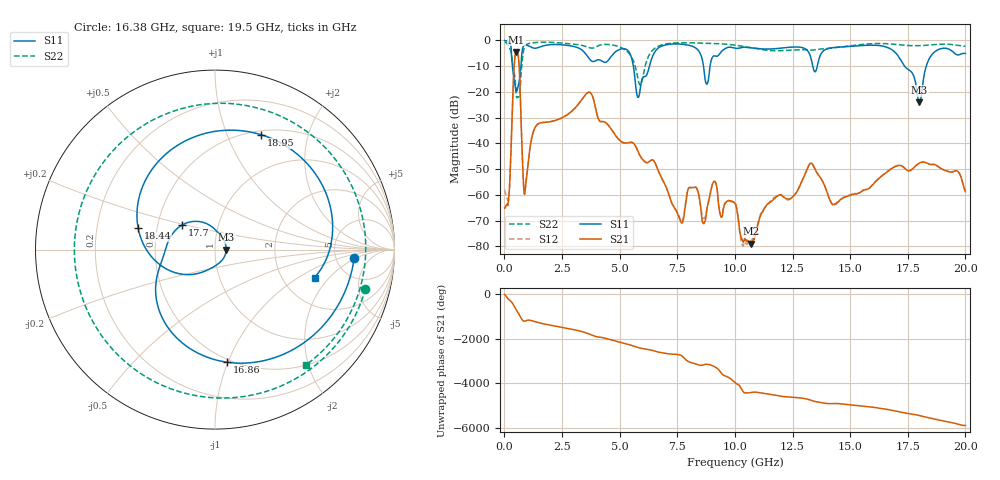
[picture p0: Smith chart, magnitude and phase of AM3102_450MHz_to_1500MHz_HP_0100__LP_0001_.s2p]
!Agilent Technologies,E8364B,MY43040894,A.07.50.67
!Agilent E8364B: A.07.50.67
!Date: Thursday, January 11, 2018 05:34:59
!Correction: S11(Full 2 Port(1,2))
!S21(Full 2 Port(1,2))
!S12(Full 2 Port(1,2))
!S22(Full 2 Port(1,2))
!S2P File: Measurements: S11, S21, S12, S22:
# Hz S  dB  R 50
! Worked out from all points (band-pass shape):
!   1601 points, 10 MHz to 20 GHz, reference 50 ohm
!   highest |S21| = -4.51 dB at 522.2 MHz (marker M1); lowest = -78.9 dB at 10.72 GHz (marker M2)
!   |S21| within 3 dB of the highest: 447.1 MHz to 622.3 MHz (175.2 MHz wide, 32.8 % of centre)
!   lowest |S11| = -24.0 dB at 18 GHz (marker M3), VSWR 1.13, Z = 56.7 + j0.0046 ohm
!   |S11| at or under -10 dB: 347.8 MHz to 720.8 MHz (372.9 MHz wide, 69.8 % of centre); 5.594 GHz to 6.296 GHz (701.5 MHz wide, 11.8 % of centre); 17.35 GHz to 18.3 GHz (949.1 MHz wide, 5.32 % of centre)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
!   |S22| runs from -22.3 to -0.6 dB; largest |S21 - S12| = 0.0028
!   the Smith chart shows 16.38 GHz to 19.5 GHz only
!   S11 on the Smith chart (normalised r, x): 16.38 GHz: 7.52, -1.79; 16.86 GHz: 0.48, -0.99; 17.7 GHz: 0.67, +0.19; 18.44 GHz: 0.39, +0.12; 18.95 GHz: 0.55, +1.33; 19.5 GHz: 3.00, -1.40
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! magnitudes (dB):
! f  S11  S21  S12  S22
! 10 MHz  -0.1  -65.0  -58.0  -0.6
! 197.4 MHz  -0.7  -60.4  -60.4  -2.7
! 522.2 MHz  -18.6  -4.5  -4.5  -21.8
! 897.1 MHz  -1.9  -58.4  -58.5  -2.2
! 1.384 GHz  -3.0  -33.1  -33.1  -0.9
! 3.346 GHz  -3.7  -23.2  -23.2  -1.9
! 5.807 GHz  -22.2  -43.3  -43.4  -15.5
! 6.682 GHz  -3.0  -50.7  -50.7  -2.3
! 7.669 GHz  -1.5  -70.7  -70.1  -1.0
! 10.01 GHz  -3.1  -63.3  -63.1  -1.9
! 10.72 GHz  -3.0  -78.9  -77.4  -2.9
! 13.34 GHz  -8.4  -47.8  -47.9  -3.8
! 14.3 GHz  -2.8  -63.7  -64.1  -2.9
! 16.38 GHz  -2.2  -52.6  -52.6  -1.3
! 16.68 GHz  -3.0  -50.6  -50.4  -1.4
! 16.86 GHz  -4.0  -49.4  -49.3  -1.5
! 17.7 GHz  -12.8  -50.0  -50.0  -2.1
! 18 GHz  -24.0  -47.7  -47.7  -2.1
! 18.44 GHz  -7.0  -48.1  -48.1  -1.8
! 18.95 GHz  -3.2  -49.8  -49.8  -1.5
! 19.5 GHz  -4.8  -50.9  -51.0  -1.7
! 20 GHz  -5.1  -58.8  -58.3  -2.4
